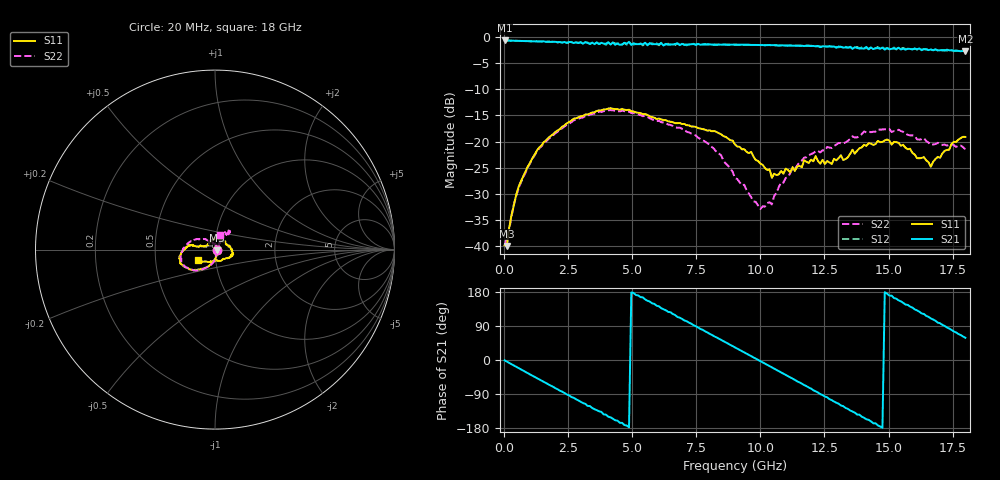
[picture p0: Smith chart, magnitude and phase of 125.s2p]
!Agilent Technologies,N5230A,US43500223,A.07.50.48
!Agilent N5230A: A.07.50.48
!Date: Sunday, January 17, 2016 20:58:42
!Correction: S11(Full 2 Port(1,2))
!S21(Full 2 Port(1,2))
!S12(Full 2 Port(1,2))
!S22(Full 2 Port(1,2))
!S2P File: Measurements: S11, S21, S12, S22:
# Hz S  RI  R 50
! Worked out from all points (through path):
!   201 points, 20 MHz to 18 GHz, reference 50 ohm
!   highest |S21| = -0.65 dB at 20 MHz (marker M1); lowest = -2.7 dB at 18 GHz (marker M2)
!   group delay of S21, straight-line fit = 102 ps
!   lowest |S11| = -40.0 dB at 109.9 MHz (marker M3), VSWR 1.02, Z = 51 - j0.354 ohm
!   |S11| at or under -10 dB: start of sweep to end of sweep
!   |S22| runs from -40.0 to -14.0 dB; largest |S21 - S12| = 0.039
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2e7  0.0102 -6.69e-05  0.9275 -0.0138  0.9276 -0.0139  0.01 -0.000414
1.099e8  0.00943 -0.00348  0.9222 -0.0705  0.9238 -0.0706  0.0113 -0.00436
4.695e8  0.00894 -0.0295  0.8752 -0.2805  0.8758 -0.2812  0.00902 -0.0287
1.0988e9  -0.012 -0.068  0.6857 -0.5978  0.6861 -0.5969  -0.00732 -0.0678
2.1776e9  -0.077 -0.107  0.1411 -0.8856  0.1414 -0.8854  -0.0683 -0.1086
3.0766e9  -0.1368 -0.1106  -0.346 -0.7916  -0.3468 -0.7995  -0.1294 -0.1104
3.7958e9  -0.1789 -0.0865  -0.6444 -0.6024  -0.6309 -0.5888  -0.1697 -0.0904
4.515e9  -0.1939 -0.0546  -0.8161 -0.2091  -0.8547 -0.2125  -0.1882 -0.0489
4.8746e9  -0.1985 -0.0377  -0.8993 -0.0375  -0.8821 -0.0567  -0.1919 -0.0285
6.0433e9  -0.1659 0.00971  -0.6701 0.5304  -0.6481 0.5245  -0.1544 0.0322
7.3918e9  -0.1369 0.0258  -0.0247 0.8566  -0.0393 0.8624  -0.1017 0.0586
9.01e9  -0.0924 0.0163  0.7061 0.4623  0.7067 0.462  -0.0224 0.039
9.9989e9  -0.0592 0.0174  0.8368 -0.044  0.8376 -0.0422  0.00842 0.0211
1.04484e10  -0.039 0.0227  0.7874 -0.28  0.7849 -0.2801  0.0124 0.0218
1.12575e10  -0.0197 0.0535  0.5383 -0.6271  0.5377 -0.6277  0.0322 0.0456
1.20666e10  0.0116 0.0637  0.1437 -0.8099  0.1536 -0.8066  0.0401 0.0664
1.30555e10  0.0543 0.0438  -0.3479 -0.7339  -0.348 -0.7171  0.0508 0.0827
1.37747e10  0.0802 0.0162  -0.6356 -0.4639  -0.6455 -0.4808  0.0594 0.0923
1.50333e10  0.0964 -0.034  -0.7511 0.1344  -0.7609 0.1302  0.0818 0.1034
1.57525e10  0.0699 -0.0476  -0.6367 0.4396  -0.6265 0.4489  0.0733 0.0901
1.66515e10  0.00836 -0.0569  -0.2556 0.7169  -0.2474 0.7161  0.0484 0.0796
1.8e10  -0.0929 -0.0606  0.3808 0.6236  0.3869 0.6264  0.0273 0.0797
